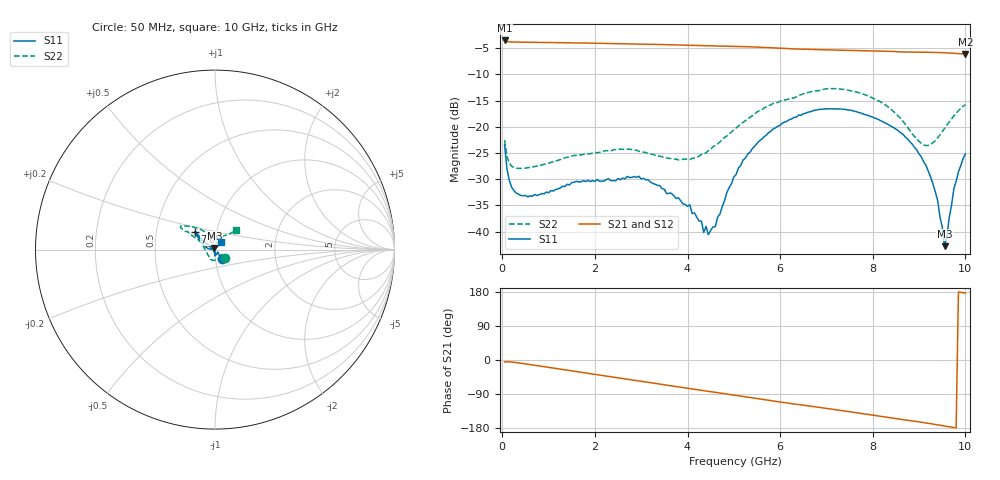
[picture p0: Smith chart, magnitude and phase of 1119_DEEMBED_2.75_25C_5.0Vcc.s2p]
!Hittite Microwave Corp.
!Digital Attenuator/PhaseShifter Rev 1.4.0
!Filename: C:\DATA\DATA\1119_DEEMBED_2.75_25C_5.0Vcc.s2p
!VNA ID: Agilent Technologies,N5224A,MY51441122,A.10.45.03
!Device type:
!2 Port Calibration.
!Temp(C): 25
!Lot Number:
!Serial Number:
!Operator:
!Misc:
!Attenuator:  2.750
# GHZ S DB R 50.0
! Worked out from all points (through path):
!   200 points, 50 MHz to 10 GHz, reference 50 ohm
!   highest |S21| = -3.54 dB at 50 MHz (marker M1); lowest = -6.1 dB at 10 GHz (marker M2)
!   group delay of S21, straight-line fit = 50 ps
!   lowest |S11| = -42.8 dB at 9.55 GHz (marker M3), VSWR 1.01, Z = 49.6 + j0.621 ohm
!   |S11| at or under -10 dB: start of sweep to end of sweep
!   |S22| runs from -28.0 to -12.7 dB; largest |S21 - S12| = 0.0017
!   S11 on the Smith chart (normalised r, x): 50 MHz: 1.07, -0.12; 7.05 GHz: 0.79, +0.16; 10 GHz: 1.07, +0.09
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0.05  -23.45 -54.5  -3.54 -5.2  -3.54 -5.2  -22.55 -40.4
0.1  -27.99 -53.2  -3.75 -4.5  -3.75 -4.5  -25.64 -35.4
0.15  -30.17 -49.3  -3.80 -4.7  -3.80 -4.7  -26.91 -31.1
0.4  -33.11 -41.3  -3.87 -8.4  -3.87 -8.5  -27.96 -28.5
1.75  -30.27 -87.0  -4.03 -33.4  -4.03 -33.4  -25.27 -73.8
2.95  -29.44 -92.2  -4.25 -55.2  -4.26 -55.2  -24.70 -114.9
3.4  -31.22 -94.0  -4.30 -63.5  -4.31 -63.6  -25.61 -129.7
4.05  -34.89 -94.8  -4.45 -75.4  -4.46 -75.5  -26.24 -160.8
4.45  -40.59 -142.5  -4.56 -82.7  -4.57 -82.8  -24.56 173.7
4.6  -39.05 -171.5  -4.58 -85.4  -4.60 -85.5  -23.60 164.7
5.05  -29.10 149.9  -4.67 -93.6  -4.69 -93.6  -20.23 151.2
5.2  -26.34 146.8  -4.71 -96.4  -4.73 -96.4  -19.14 149.4
5.75  -21.12 143.1  -4.91 -106.5  -4.92 -106.6  -16.00 147.9
6.7  -16.98 138.5  -5.25 -122.7  -5.26 -122.7  -13.26 147.5
7.05  -16.58 138.4  -5.34 -128.6  -5.35 -128.6  -12.73 146.3
8.35  -19.65 146.7  -5.62 -151.8  -5.62 -151.8  -16.34 128.4
8.75  -22.32 155.0  -5.77 -158.9  -5.77 -158.9  -20.09 116.3
9.15  -27.42 170.3  -5.79 -166.1  -5.80 -166.1  -23.61 94.4
9.400001  -34.02 171.6  -5.82 -171.1  -5.84 -171.1  -22.16 66.7
9.55  -42.79 120.4  -5.88 -174.2  -5.89 -174.2  -20.29 54.5
9.75  -31.87 51.4  -5.98 -178.3  -5.99 -178.3  -17.95 46.0
10  -25.18 51.4  -6.13 176.6  -6.14 176.6  -15.78 42.6
